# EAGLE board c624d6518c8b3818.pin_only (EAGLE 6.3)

Size 30.48 x 21.59 mm. Coordinates in mm from the lower left corner, seen from the top.
Outline: 0,2.54 0,19.05 arc-90 2.54,21.59 27.94,21.59 arc-90 30.48,19.05 30.48,2.54 arc-90 27.94,0 2.54,0 arc-90 0,2.54
Copper layers (1*16): Top 0.035mm / dielectric 1.5mm / Bottom 0.035mm
Design rules "adafruit": minimum track width 8mil, minimum drill 15.5mil, track to track 8mil, track to pad 8mil, pad to pad 8mil, via to via 8mil, smd to smd 8mil, copper to edge 10mil, drill to drill 8mil, minimum pad ring 10mil, minimum via ring 8mil, stop-mask expansion 2mil, vias tented up to drill 20mil, thermal gap 10mil

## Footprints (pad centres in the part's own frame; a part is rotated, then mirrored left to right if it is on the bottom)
0805-NO = smd 1.3 x 1.5: 1 -0.95,0; 2 0.95,0
FIDUCIAL_1MM = smd 1 x 1: 1 0,0
1X07_ROUND_76 = drill 1 pad 1.93 square: 1 -7.62,0 | drill 1 pad 1.93: 2 -5.08,0; 3 -2.54,0; 4 0,0; 5 2.54,0; 6 5.08,0; 7 7.62,0
SOT23-WIDE = smd 1 x 1.2: 1 -0.95,-1; 2 0.95,-1; 3 0,1
MSOP10 = smd 0.25 x 1: 1 -1,-2.113; 2 -0.5,-2.113; 3 0,-2.113; 4 0.5,-2.113; 5 1,-2.113; 6 1,2.113; 7 0.5,2.113; 8 0,2.113; 9 -0.5,2.113; 10 -1,2.113
SOT23-5 = smd 0.55 x 1.2: 1 -0.95,-1.3; 2 0,-1.3; 3 0.95,-1.3; 4 0.95,1.3; 5 -0.95,1.3
MOUNTINGHOLE_2.5_PLATED = drill 2.5 pad 3.2: P$1 0,0
SMA_EDGELAUNCH = smd 4.064 x 1.524: GND@1 2.032,-2.54; GND@2 2.032,2.54 | smd 4.064 x 1.524 bottom: GND@3 2.032,2.54; GND@4 2.032,-2.54 | smd 4.064 x 1.27: P 2.032,0
CRYSTAL_3.2X2.5 = smd 1.4 x 1.2: 1 -1.1,-0.8; 2 1.1,0.8; GND1 -1.1,0.8; GND2 1.1,-0.8

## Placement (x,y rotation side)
C1  0.47uF  [0805-NO]  12.7,11.94 90 top
C2  0.47uF  [0805-NO]  19.56,13.72 180 top
C3  10µF  [0805-NO]  27.69,12.19 180 top
C5  10µF  [0805-NO]  27.43,6.6 0 top
FID1  FIDUCIAL""  [FIDUCIAL_1MM]  28.96,14.48 180 top
FID2  FIDUCIAL""  [FIDUCIAL_1MM]  5.59,1.27 180 top
JP1  [1X07_ROUND_76]  15.24,2.54 180 top
Q1  BSS138  [SOT23-WIDE]  23.62,11.18 180 top
Q2  BSS138  [SOT23-WIDE]  19.56,8.89 180 top
R5  10K  [0805-NO]  19.56,11.68 0 top
R6  10K  [0805-NO]  23.62,13.97 0 top
R7  10K  [0805-NO]  23.62,7.37 270 top
R8  10K  [0805-NO]  20.32,5.84 0 top
U1  Si5351A-B-GT  [MSOP10]  15.49,12.19 0 top
U2  RT9193  [SOT23-5]  27.43,9.4 270 top
U$10  MOUNTINGHOLE2.5  [MOUNTINGHOLE_2.5_PLATED]  27.94,2.54 180 top
U$11  MOUNTINGHOLE2.5  [MOUNTINGHOLE_2.5_PLATED]  2.54,2.54 180 top
U$12  [ADAFRUIT_3.5MM]  0.51,10.67 0 top
U$23  [ADAFRUIT_TEXT_20MM]  26.16,4.32 0 bottom
X1  [SMA_EDGELAUNCH]  5.08,21.08 270 top
X2  [SMA_EDGELAUNCH]  15.24,21.08 270 top
X3  [SMA_EDGELAUNCH]  25.4,21.08 270 top
Y1  25MHz  [CRYSTAL_3.2X2.5]  15.24,7.37 180 top

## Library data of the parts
C1-C3 C5 JP1 Q1 Q2 R5-R8 U1 U2 U$12 U$23 X1-X3 Y1 = microbuilder
FID1 FID2 U$10 U$11 = microbuilder; BOM: EXCLUDE

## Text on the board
tPlace: CLK0 | CLK1 | CLK2 | SI5351 / Clock Gen | 25MHz Xtal / 8kHz-160 MHz | 1 | SCL | GND | 0 | 2 | SDA | VIN
bPlace: Si5351 8 kHz - 160 MHz / Clock Generator | Vin: 3.3V - 5V / Logic: 3.3-5V

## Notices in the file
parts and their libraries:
microbuilder: This work is placed in the public domain, and may be freely used for commercial and non-commercial work with the following conditions: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
